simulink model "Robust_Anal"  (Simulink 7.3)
settings: Solver=ode45  StartTime=0.0  StopTime=30  RelTol=1e-3
InitFcn:
  | start
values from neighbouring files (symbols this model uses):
  d2r = pi/180    (= 0.0174532925199)    [start.m]    (also in Pl.m; run.m; pl.m)
  Ka = (1+2*zeta*lamb)*Jgi*wcmg^2    (= 292500)    [start.m]
  Kb = (2*zeta+lamb)*wcmg/Ka    (= 0.00410256410256)    [start.m]
  ki = 0.07    [start.m]
  Kii = lamb*Jgi*wcmg^3    (= 37500000)    [start.m]
  kp = 7.3    [start.m]
  r2d = 180/pi    (= 57.2957795131)    [start.m]    (also in Pl.m; run.m; pl.m)
undefined symbols (not defined in the file or in its folder): Au, Bu, Cu, Du, Lin_Steering, Tglim

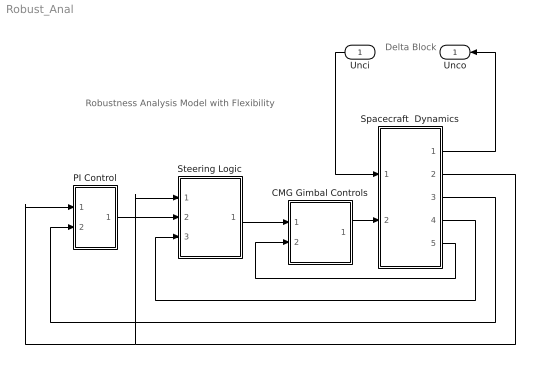
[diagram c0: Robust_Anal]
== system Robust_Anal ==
  note: Robustness Analysis Model with Flexibility
  note: Delta Block
  Unci : Inport  OutDataType=sfix(16)  OutScaling=2^0
  CMG Gimbal Controls : Subsystem
  PI Control : Subsystem
  Spacecraft  Dynamics : Subsystem
  Steering Logic : Subsystem
  Unco : Outport  OutDataType=sfix(16)  OutScaling=2^0
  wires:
  CMG Gimbal Controls/1(Tc) -> Spacecraft  Dynamics/2(Tc)
  Spacecraft  Dynamics/5(deldot) -> CMG Gimbal Controls/2(deldot)
  Steering Logic/1(deldot) -> CMG Gimbal Controls/1(deldc)
  Spacecraft  Dynamics/2(rate) -> Steering Logic/1(wb), PI Control/1(wb)
  Spacecraft  Dynamics/4(delta) -> Steering Logic/3(delta)
  PI Control/1(wer) -> Steering Logic/2(we)
  Spacecraft  Dynamics/3(atti) -> PI Control/2(ater)
  Unci/1 -> Spacecraft  Dynamics/1(Unci)
  Spacecraft  Dynamics/1(Unco) -> Unco/1

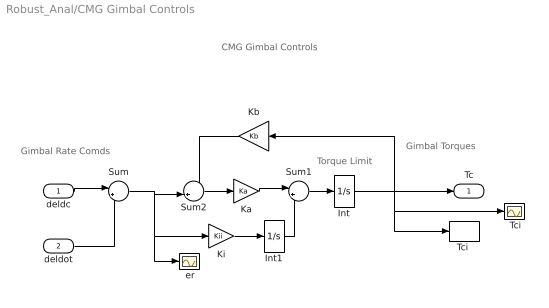
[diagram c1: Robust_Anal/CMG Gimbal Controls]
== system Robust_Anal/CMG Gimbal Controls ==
  note: Gimbal Rate Comds
  note: CMG Gimbal Controls
  note: Torque Limit
  note: Gimbal Torques
  deldc : Inport  PortDimensions=4  OutDataType=sfix(16)  OutScaling=2^0
  deldot : Inport  Port=2  PortDimensions=4  OutDataType=sfix(16)  OutScaling=2^0
  " Tci" : Scope
  " er" : Scope
  Int : Integrator  UpperSaturationLimit=[1 1 1 1]*Tglim  LowerSaturationLimit=-[1 1 1 1]*Tglim
  Int1 : Integrator  UpperSaturationLimit=0  LowerSaturationLimit=0
  Ka : Gain  Gain=Ka  ParameterDataType=sfix(16)  ParameterScaling=2^0  OutDataType=sfix(16)  OutScaling=2^0
  Kb : Gain  Gain=Kb  ParameterDataType=sfix(16)  ParameterScaling=2^0  OutDataType=sfix(16)  OutScaling=2^0
  Ki : Gain  Gain=Kii  ParameterDataType=sfix(16)  ParameterScaling=2^0  OutDataType=sfix(16)  OutScaling=2^0
  Sum : Sum  Inputs=|+-  OutDataType=sfix(16)  OutScaling=2^0
  Sum1 : Sum  Inputs=|++  OutDataType=sfix(16)  OutScaling=2^0
  Sum2 : Sum  Inputs=-+|  OutDataType=sfix(16)  OutScaling=2^0
  "Tci " : ToWorkspace  VariableName=Tci  SampleTime=-1  SaveFormat=Array
  Tc : Outport  OutDataType=sfix(16)  OutScaling=2^0
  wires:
  deldot/1 -> Sum/2
  deldc/1 -> Sum/1
  Sum/1 -> " er"/1, Ki/1, Sum2/2
  Kb/1 -> Sum2/1
  Int1/1 -> Sum1/2
  Ki/1 -> Int1/1
  Sum1/1 -> Int/1
  Ka/1 -> Sum1/1
  Sum2/1 -> Ka/1
  Int/1 -> Tc/1, " Tci"/1, "Tci "/1, Kb/1

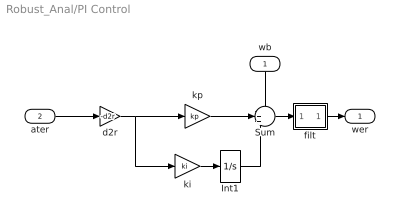
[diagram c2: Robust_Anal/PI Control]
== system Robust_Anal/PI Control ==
  wb : Inport
  ater : Inport  Port=2
  Int1 : Integrator  UpperSaturationLimit=0  LowerSaturationLimit=0
  Sum : Sum  Inputs=-++  OutDataType=sfix(16)  OutScaling=2^0
  d2r : Gain  Gain=-d2r  ParameterDataType=sfix(16)  ParameterScaling=2^0  OutDataType=sfix(16)  OutScaling=2^0
  filt : Subsystem
  ki : Gain  Gain=ki  ParameterDataType=sfix(16)  ParameterScaling=2^0  OutDataType=sfix(16)  OutScaling=2^0
  kp : Gain  Gain=kp  ParameterDataType=sfix(16)  ParameterScaling=2^0  OutDataType=sfix(16)  OutScaling=2^0
  wer : Outport
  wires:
  ater/1 -> d2r/1
  kp/1 -> Sum/2
  ki/1 -> Int1/1
  Int1/1 -> Sum/3
  wb/1 -> Sum/1
  Sum/1 -> filt/1(in)
  d2r/1 -> ki/1, kp/1
  filt/1(ou) -> wer/1

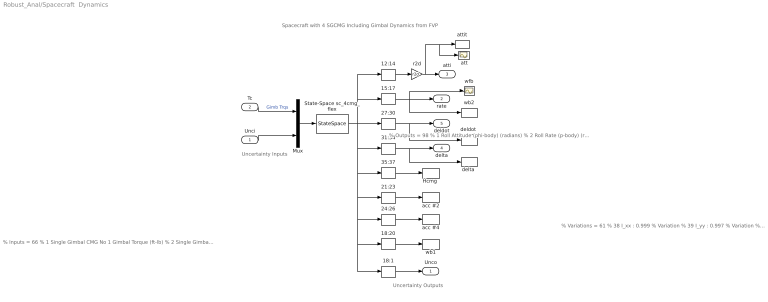
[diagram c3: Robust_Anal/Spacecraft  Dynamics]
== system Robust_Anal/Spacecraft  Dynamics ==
  note: Spacecraft with 4 SGCMG Including Gimbal Dynamics from FVP
  note: % Outputs = 98 % 1 Roll Attitude (phi-body) (radians) % 2 Roll Rate (p-body) (rad/sec) % 3 Pitch Attitude (thet-bdy) (radians) % 4 Pitch Rate (q-body) (rad/sec) % 5 Yaw Attitude (psi-body) (radians) % 6 Yaw Rate (r-body) (rad/sec) % 7 Angle of attack, alfa, (radians) % 8 Angle of sideslip, beta, (radian) % 9 Change in Altitude, delta-h, (feet) % 10 Forward Acceleration (V-dot) (ft/sec) % 11 Cross Range Velocity (Vcr) (ft/sec) % 12 Gyro # 1, Roll Attitude (Body) (radians) % 13 Gyro # 2, Pitch Attitude (Body) (radians) % 14 Gyro # 3, Yaw Attitude (Body) (radians) % 15 Rate-Gyro # 4, Roll Rate (Body) (rad/sec) % 16 Rate-Gyro # 5, Pitch Rate (Body) (rad/sec) % 17 Rate-Gyro # 6, Yaw Rate (Body) (rad/sec) % 18 Rate-Gyro # 7, Roll Rate (Body) (rad/sec) % 19 Rate-Gyro # 8, Pitch Rate (Body) (rad/sec) % 20 Rate-Gyro # 9, Yaw Rate (Body) (rad/sec) % 21 Accelerom # 1, (along X), (ft/sec^2) Translat. Acceler % 22 Accelerom # 2, (along Y), (ft/sec^2) Translat. Acceler % 23 Accelerom # 3, (along Z), (ft/sec^2) Translat. Acceler % 24 Accelerom # 4, (along X), (ft/sec^2) Translat. Acceler % 25 Accelerom # 5, (along Y), (ft/sec^2) Translat. Acceler % 26 Accelerom # 6, (along Z), (ft/sec^2) Translat. Acceler % 27 SGCMG # 1 Gimbal Rate (rad/sec) % 28 SGCMG # 2 Gimbal Rate (rad/sec) % 29 SGCMG # 3 Gimbal Rate (rad/sec) % 30 SGCMG # 4 Gimbal Rate (rad/sec) % 31 SGCMG # 1 Gimbal Angle (radian) % 32 SGCMG # 2 Gimbal Angle (radian) % 33 SGCMG # 3 Gimbal Angle (radian) % 34 SGCMG # 4 Gimbal Angle (radian) % 35 SGCMG Array Momentum in X-axis (ft-lb-sec) % 36 SGCMG Array Momentum in Y-axis (ft-lb-sec) % 37 SGCMG Array Momentum in Z-axis (ft-lb-sec)
  note: % Variations = 61 % 38 I_xx : 0.999 % Variation % 39 I_yy : 0.997 % Variation % 40 I_zz : 0.966 % Variation % 41 I_xz : 0.994 % Variation % 42 I_xz : 0.994 % Variation % 43 I_yz : 0.997 % Variation % 44 I_yz : 0.997 % Variation % 45 I_xy : 0.999 % Variation % 46 I_xy : 0.999 % Variation % 47 Jgimbl- 1: 10.000 % Variation % 48 H0cmg - 1: 3.333 % Variation % 49 H0cmg - 1: 3.333 % Variation % 50 Delta0- 1: 0.8727E-02 Addit. Variat. % 51 Delta0- 1: 0.8727E-02 Addit. Variat. % 52 Beta - 1: 0.735 % Variation % 53 Beta - 1: 0.735 % Variation % 54 Gamma - 1: 0.556 % Variation % 55 Gamma - 1: 0.556 % Variation % 56 HDirect 1: 14.003 % Variation % 57 HDirect 1: 14.003 % Variation % 58 Jgimbl- 2: 10.000 % Variation % 59 H0cmg - 2: 3.333 % Variation % 60 H0cmg - 2: 3.333 % Variation % 61 Delta0- 2: 0.8727E-02 Addit. Variat. % 62 Delta0- 2: 0.8727E-02 Addit. Variat. % 63 Beta - 2: 0.735 % Variation % 64 Beta - 2: 0.735 % Variation % 65 Gamma - 2: 0.278 % Variation % 66 Gamma - 2: 0.278 % Variation % 67 HDirect 2: 14.003 % Variation % 68 HDirect 2: 14.003 % Variation % 69 Jgimbl- 3: 10.000 % Variation % 70 H0cmg - 3: 3.333 % Variation % 71 H0cmg - 3: 3.333 % Variation % 72 Delta0- 3: 0.8727E-02 Addit. Variat. % 73 Delta0- 3: 0.8727E-02 Addit. Variat. % 74 Beta - 3: 0.735 % Variation % 75 Beta - 3: 0.735 % Variation % 76 Gamma - 3: 0.185 % Variation % 77 Gamma - 3: 0.185 % Variation % 78 HDirect 3: 14.003 % Variation % 79 HDirect 3: 14.003 % Variation % 80 Jgimbl- 4: 10.000 % Variation % 81 H0cmg - 4: 3.333 % Variation % 82 H0cmg - 4: 3.333 % Variation % 83 Delta0- 4: 0.8727E-02 Addit. Variat. % 84 Delta0- 4: 0.8727E-02 Addit. Variat. % 85 Beta - 4: 0.735 % Variation % 86 Beta - 4: 0.735 % Variation % 87 Gamma - 4: 0.8727E-02 Addit. Variat. % 88 Gamma - 4: 0.8727E-02 Addit. Variat. % 89 HDirect 4: 14.003 % Variation % 90 HDirect 4: 14.003 % Variation % 91 W_flex 1: 0.4000 Addit. Variat. % 92 W_flex 2: 0.7000 Addit. Variat. % 93 W_flex 3: 1.200 Addit. Variat. % 94 W_flex 4: 3.000 A
  note: % Inputs = 66 % 1 Single Gimbal CMG No 1 Gimbal Torque (ft-lb) % 2 Single Gimbal CMG No 2 Gimbal Torque (ft-lb) % 3 Single Gimbal CMG No 3 Gimbal Torque (ft-lb) % 4 Single Gimbal CMG No 4 Gimbal Torque (ft-lb) % 5 Ext Force Direct.=( 1.0000 0.0000 0.0000) % 6 I_xx : 0.999 % Variation % 7 I_yy : 0.997 % Variation % 8 I_zz : 0.966 % Variation % 9 I_xz : 0.994 % Variation % 10 I_xz : 0.994 % Variation % 11 I_yz : 0.997 % Variation % 12 I_yz : 0.997 % Variation % 13 I_xy : 0.999 % Variation % 14 I_xy : 0.999 % Variation % 15 Jgimbl- 1: 10.000 % Variation % 16 H0cmg - 1: 3.333 % Variation % 17 H0cmg - 1: 3.333 % Variation % 18 Delta0- 1: 0.8727E-02 Addit. Variat. % 19 Delta0- 1: 0.8727E-02 Addit. Variat. % 20 Beta - 1: 0.735 % Variation % 21 Beta - 1: 0.735 % Variation % 22 Gamma - 1: 0.556 % Variation % 23 Gamma - 1: 0.556 % Variation % 24 HDirect 1: 14.003 % Variation % 25 HDirect 1: 14.003 % Variation % 26 Jgimbl- 2: 10.000 % Variation % 27 H0cmg - 2: 3.333 % Variation % 28 H0cmg - 2: 3.333 % Variation % 29 Delta0- 2: 0.8727E-02 Addit. Variat. % 30 Delta0- 2: 0.8727E-02 Addit. Variat. % 31 Beta - 2: 0.735 % Variation % 32 Beta - 2: 0.735 % Variation % 33 Gamma - 2: 0.278 % Variation % 34 Gamma - 2: 0.278 % Variation % 35 HDirect 2: 14.003 % Variation % 36 HDirect 2: 14.003 % Variation % 37 Jgimbl- 3: 10.000 % Variation % 38 H0cmg - 3: 3.333 % Variation % 39 H0cmg - 3: 3.333 % Variation % 40 Delta0- 3: 0.8727E-02 Addit. Variat. % 41 Delta0- 3: 0.8727E-02 Addit. Variat. % 42 Beta - 3: 0.735 % Variation % 43 Beta - 3: 0.735 % Variation % 44 Gamma - 3: 0.185 % Variation % 45 Gamma - 3: 0.185 % Variation % 46 HDirect 3: 14.003 % Variation % 47 HDirect 3: 14.003 % Variation % 48 Jgimbl- 4: 10.000 % Variation % 49 H0cmg - 4: 3.333 % Variation % 50 H0cmg - 4: 3.333 % Variation % 51 Delta0- 4: 0.8727E-02 Addit. Variat. % 52 Delta0- 4: 0.8727E-02 Addit. Variat. % 53 Beta - 4: 0.735 % Variation % 54 Beta - 4: 0.735 % Variation % 55 Gamma - 4: 0.8727E-02 Addit. Variat. % 56 Gamma
  note: Uncertainty Inputs
  note: Uncertainty Outputs
  Unci : Inport  OutDataType=sfix(16)  OutScaling=2^0
  Tc : Inport  Port=2  PortDimensions=4  OutDataType=sfix(16)  OutScaling=2^0
  " att" : Scope
  " wfb " : Scope
  12:14 : Selector  InputPortWidth=98  IndexOptions=Index vector (dialog)  Indices=[12:14]  OutputSizes=1
  15:17 : Selector  InputPortWidth=98  IndexOptions=Index vector (dialog)  Indices=[15:17]  OutputSizes=1
  18:1 : Selector  InputPortWidth=98  IndexOptions=Index vector (dialog)  Indices=[38:98]  OutputSizes=1
  18:20 : Selector  InputPortWidth=98  IndexOptions=Index vector (dialog)  Indices=[18:20]  OutputSizes=1
  21:23 : Selector  InputPortWidth=98  IndexOptions=Index vector (dialog)  Indices=[21:23]  OutputSizes=1
  24:26 : Selector  InputPortWidth=98  IndexOptions=Index vector (dialog)  Indices=[24:26]  OutputSizes=1
  27:30 : Selector  InputPortWidth=98  IndexOptions=Index vector (dialog)  Indices=[27:30]  OutputSizes=1
  31:34 : Selector  InputPortWidth=98  IndexOptions=Index vector (dialog)  Indices=[31:34]  OutputSizes=1
  35:37 : Selector  InputPortWidth=98  IndexOptions=Index vector (dialog)  Indices=[35:37]  OutputSizes=1
  "Hcmg " : ToWorkspace  VariableName=Hcmg  SampleTime=-1  SaveFormat=Array
  Mux : Mux  Inputs="[4,  1, 61]"
  State-Space sc_4cmg_flex : StateSpace  A=Au  B=Bu  C=Cu  D=Du
  acc #2 : ToWorkspace  VariableName=acc_2  SampleTime=-1  SaveFormat=Array
  acc #4 : ToWorkspace  VariableName=acc_4  SampleTime=-1  SaveFormat=Array
  attit : ToWorkspace  VariableName=atti  SampleTime=-1  SaveFormat=Array
  "deldot " : ToWorkspace  VariableName=deld  SampleTime=-1  SaveFormat=Array
  "delta " : ToWorkspace  VariableName=delta  SampleTime=-1  SaveFormat=Array
  r2d : Gain  Gain=r2d  ParameterDataType=sfix(16)  ParameterScaling=2^0  OutDataType=sfix(16)  OutScaling=2^0
  wb1 : ToWorkspace  VariableName=wb_1  SampleTime=-1  SaveFormat=Array
  wb2 : ToWorkspace  VariableName=wb_2  SampleTime=-1  SaveFormat=Array
  Unco : Outport  OutDataType=sfix(16)  OutScaling=2^0
  rate : Outport  Port=2  OutDataType=sfix(16)  OutScaling=2^0
  atti : Outport  Port=3  OutDataType=sfix(16)  OutScaling=2^0
  delta : Outport  Port=4  OutDataType=sfix(16)  OutScaling=2^0
  deldot : Outport  Port=5  OutDataType=sfix(16)  OutScaling=2^0
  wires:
  Mux/1 -> State-Space sc_4cmg_flex/1
  Tc/1 -> Mux/1  "Gimb Trqs"
  State-Space sc_4cmg_flex/1 -> 12:14/1, 15:17/1, 27:30/1, 31:34/1, 35:37/1, 21:23/1, 24:26/1, 18:20/1, 18:1/1
  12:14/1 -> r2d/1
  15:17/1 -> rate/1, wb2/1, " wfb "/1
  27:30/1 -> deldot/1, "deldot "/1
  31:34/1 -> delta/1, "delta "/1
  35:37/1 -> "Hcmg "/1
  r2d/1 -> atti/1, attit/1, " att"/1
  18:20/1 -> wb1/1
  21:23/1 -> acc #2/1
  24:26/1 -> acc #4/1
  Unci/1 -> Mux/3
  18:1/1 -> Unco/1

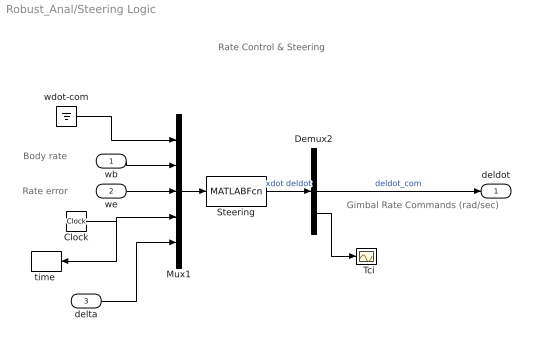
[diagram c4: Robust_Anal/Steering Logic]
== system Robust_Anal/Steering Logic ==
  note: Body rate
  note: Rate error
  note: Gimbal Rate Commands (rad/sec)
  note: Rate Control & Steering
  wb : Inport  PortDimensions=3  OutDataType=sfix(16)  OutScaling=2^0
  we : Inport  Port=2  PortDimensions=3  OutDataType=sfix(16)  OutScaling=2^0
  delta : Inport  Port=3  OutDataType=sfix(16)  OutScaling=2^0
  "  Tci" : Scope
  Clock : Clock
  Demux2 : Demux  Outputs=[3,4,4]
  Mux1 : Mux  Inputs=[3,3,3, 1,4]
  Steering : MATLABFcn  MATLABFcn=Lin_Steering( u(1:3), u(4:6), u(7:9), u(10), u(11:14) )  OutputDimensions=11
  "time " : ToWorkspace  VariableName=time  SampleTime=-1  SaveFormat=Array
  wdot-com : Ground
  deldot : Outport  OutDataType=sfix(16)  OutScaling=2^0
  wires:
  Demux2/3 -> "  Tci"/1
  delta/1 -> Mux1/5
  Mux1/1 -> Steering/1
  we/1 -> Mux1/3
  Clock/1 -> "time "/1, Mux1/4
  wb/1 -> Mux1/2
  Demux2/2 -> deldot/1  "deldot_com"
  Steering/1 -> Demux2/1  "xdot deldot"
  wdot-com/1 -> Mux1/1

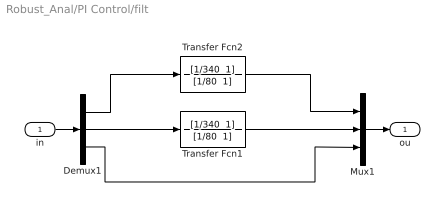
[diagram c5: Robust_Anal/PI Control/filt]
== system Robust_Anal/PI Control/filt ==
  in : Inport  OutDataType=sfix(16)  OutScaling=2^0
  Demux1 : Demux  Outputs=3
  Mux1 : Mux  Inputs=3
  Transfer Fcn1 : TransferFcn  Numerator="[1/340  1]"  Denominator="[1/80  1]"
  Transfer Fcn2 : TransferFcn  Numerator="[1/340  1]"  Denominator="[1/80  1]"
  ou : Outport  OutDataType=sfix(16)  OutScaling=2^0
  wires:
  Demux1/1 -> Transfer Fcn2/1
  Demux1/2 -> Transfer Fcn1/1
  Demux1/3 -> Mux1/3
  in/1 -> Demux1/1
  Mux1/1 -> ou/1
  Transfer Fcn2/1 -> Mux1/1
  Transfer Fcn1/1 -> Mux1/2
